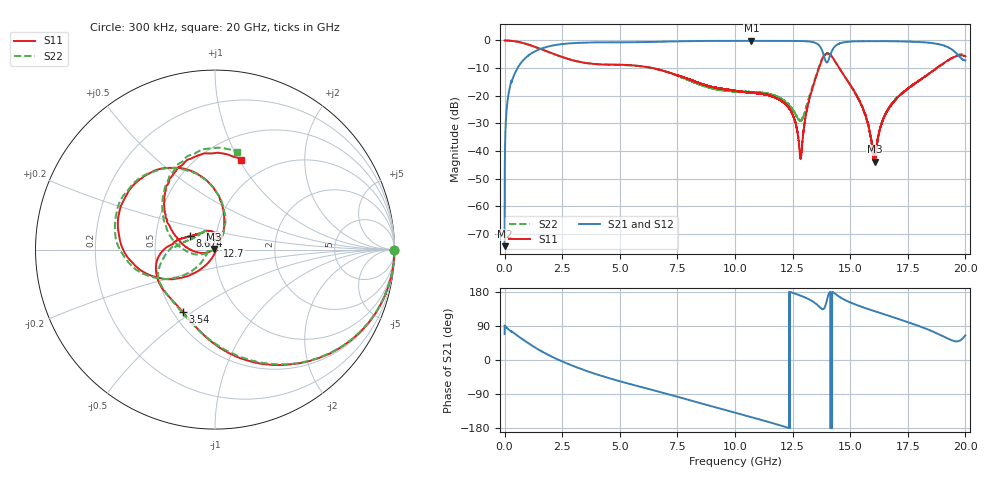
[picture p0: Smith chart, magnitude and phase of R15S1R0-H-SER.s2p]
!{R15S1R0}
!Johanson Technology Inc.
!www.johansontechnology.com
!Test Board Conditions:
!Substrate Type  RO4350B
!Substrate Thickness  20 mil
!Substrate Dk  3.66
!TL Type: GCPW
!TL Trace Width  34 mil
!TL Gap  10 mil
!Electrode orientation  Horizontal
!DUT TOPOLOGY	SERIES
!Mounting Pad LxW  26x52 mil
! Created Sat Feb  6 12:10:21 2021
# hz S ma R 50
! 2 Port Network Data from SP1.SP block
! freq  magS11  angS11  magS21  angS21  magS12  angS12  magS22  angS22
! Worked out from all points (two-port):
!   20001 points, 300 kHz to 20 GHz, reference 50 ohm
!   highest |S21| = -0.13 dB at 10.71 GHz (marker M1); lowest = -74.4 dB at 300 kHz (marker M2)
!   |S21| within 3 dB of the highest: 1.535 GHz to 13.76 GHz (12.22 GHz wide, 160 % of centre); 14.25 GHz to 19.39 GHz (5.138 GHz wide, 30.5 % of centre)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
!   lowest |S11| = -43.8 dB at 16.07 GHz (marker M3), VSWR 1.01, Z = 49.4 + j0.324 ohm
!   |S11| at or under -10 dB: 6.444477 GHz to 6.445648 GHz (1.171 MHz wide, 0.0182 % of centre); 6.454 GHz to 13.64 GHz (7.188 GHz wide, 71.5 % of centre); 14.53 GHz to 18.75 GHz (4.223 GHz wide, 25.4 % of centre)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
!   |S22| runs from -43.2 to 0.0 dB; largest |S21 - S12| = 0.014
!   S11 on the Smith chart (normalised r, x): 300 kHz: open; 3.54 GHz: 0.56, -0.46; 8.674 GHz: 0.75, +0.11; 12.7 GHz: 1.03, +0.04; 20 GHz: 0.75, +1.03
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300000  0.9974 -0.1  0.0001914 68.4  0.000175 91.2  0.997 -0.2
1.343e8  0.9954 -6.7  0.08574 82.9  0.08616 83.0  0.996 -6.7
5.153e8  0.955 -23.5  0.2929 66.1  0.2931 66.3  0.9541 -23.5
1.9613e9  0.6084 -78.7  0.7883 11.5  0.7895 11.5  0.6042 -78.0
3.3343e9  0.4043 -113.3  0.908 -24.0  0.9089 -23.9  0.4037 -114.4
3.5403e9  0.3908 -117.6  0.9136 -28.5  0.9146 -28.4  0.3902 -119.1
6.6673e9  0.3002 -176.9  0.9453 -83.2  0.9464 -83.2  0.2976 -169.0
8.6743e9  0.1582 151.7  0.9794 -116.9  0.9792 -116.8  0.1502 157.8
1.00003e10  0.1237 132.6  0.9826 -139.0  0.9832 -139.0  0.1197 131.1
1.07093e10  0.1141 118.1  0.9854 -150.8  0.9809 -150.9  0.1173 121.0
1.21563e10  0.07224 80.4  0.9791 -176.0  0.9798 -176.0  0.08064 114.9
1.27023e10  0.02334 54.9  0.9778 173.1  0.9781 173.1  0.04097 139.3
1.28763e10  0.008672 -46.8  0.975 169.1  0.975 169.2  0.03605 176.0
1.33343e10  0.1255 -124.7  0.9435 156.0  0.9447 156.0  0.1354 -136.2
1.38963e10  0.5438 170.4  0.4698 138.7  0.4695 138.2  0.5623 171.7
1.41603e10  0.5389 123.1  0.5788 -179.3  0.5788 -179.9  0.5395 124.3
1.45803e10  0.2924 85.0  0.8969 164.8  0.8925 164.8  0.2915 84.7
1.54813e10  0.06831 60.6  0.9678 140.7  0.9649 140.9  0.06832 60.4
1.60713e10  0.006467 149.5  0.9712 128.5  0.9714 128.7  0.008927 145.9
1.66673e10  0.05861 -162.5  0.9724 116.7  0.9642 116.8  0.05993 -158.0
1.91523e10  0.4123 132.9  0.7869 59.1  0.788 59.4  0.4094 135.6
2e10  0.5189 73.2  0.4376 65.1  0.4337 65.5  0.5563 76.6
